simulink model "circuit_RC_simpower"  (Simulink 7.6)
settings: Solver=ode23t  StartTime=0.0  StopTime=0.04  RelTol=1e-3
InitFcn:
  | clc, close all
StopFcn:
  | close all
  | load tension_Vc.mat
  | plot(x(1,:),x(2,:), x(1,:),x(3,:),x(1,:),x(4,:))
  | axis([0 0.04 -60 120])
  | grid
  | title('Tension aux bornes de C, courant et créneau d''entrée')
  | xlabel('temps')
libraries: powerlib x9

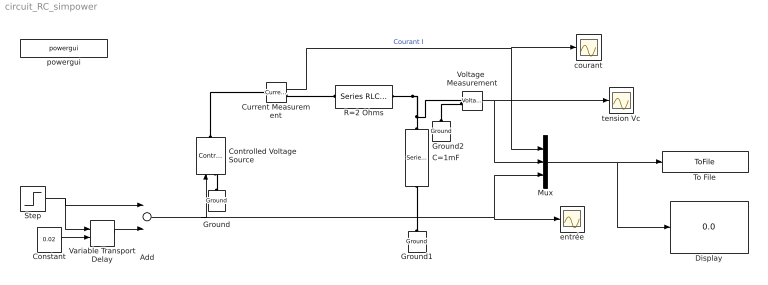
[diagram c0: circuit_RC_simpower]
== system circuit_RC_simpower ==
  Add : Sum  Inputs=+-
  C=1mF : powerlib/Elements/Series RLC Branch  DialogController=POWERSYS.PowerSysDialog  PhysicalDomain=powersysdomain  SubClassName=unknown  LeftPortType=p1  RightPortType=p1  LConnTagsString=__new0  RConnTagsString=__new0  BranchType=C  Resistance=2  Inductance=1e-3  SetiL0=off  InitialCurrent=0  Capacitance=1e-3  Setx0=off  InitialVoltage=0  Measurements=None
  Constant : Constant  Value=0.02
  Controlled Voltage Source : powerlib/Electrical Sources/Controlled Voltage Source  DialogController=POWERSYS.PowerSysDialog  SystemSampleTime=-1  Initialize=on  Source_Type=AC  Amplitude=0  Phase=0  Frequency=0  Measurements=None
  Current Measurement : powerlib/Measurements/Current Measurement  DialogController=POWERSYS.PowerSysDialog  SystemSampleTime=-1  PhasorSimulation=off  OutputType=Complex  PSBequivalent=0
  Display : Display
  Ground : powerlib/Elements/Ground  DialogController=POWERSYS.PowerSysDialog  PhysicalDomain=powersysdomain  SubClassName=unknown  LeftPortType=p1  RightPortType=p1  LConnTagsString=a
  Ground1 : powerlib/Elements/Ground  DialogController=POWERSYS.PowerSysDialog  PhysicalDomain=powersysdomain  SubClassName=unknown  LeftPortType=p1  RightPortType=p1  LConnTagsString=a
  Ground2 : powerlib/Elements/Ground  DialogController=POWERSYS.PowerSysDialog  PhysicalDomain=powersysdomain  SubClassName=unknown  LeftPortType=p1  RightPortType=p1  LConnTagsString=a
  Mux : Mux  Inputs=3
  R=2 Ohms : powerlib/Elements/Series RLC Branch  DialogController=POWERSYS.PowerSysDialog  PhysicalDomain=powersysdomain  SubClassName=unknown  LeftPortType=p1  RightPortType=p1  LConnTagsString=__new0  RConnTagsString=__new0  BranchType=R  Resistance=2  Inductance=1e-3  SetiL0=off  InitialCurrent=0  Capacitance=1e-6  Setx0=off  InitialVoltage=0  Measurements=None
  Step : Step  Time=0.005  After=100  SampleTime=0
  To File : ToFile  Filename=tension_Vc.mat  MatrixName=x
  Variable Transport Delay : VariableTransportDelay  VariableDelayType=Variable transport delay  MaximumDelay=10
  Voltage  Measurement : powerlib/Measurements/Voltage Measurement  DialogController=POWERSYS.PowerSysDialog  SystemSampleTime=-1  PhasorSimulation=off  OutputType=Complex  PSBequivalent=0
  courant : Scope
  entrée : Scope
  powergui : powerlib/powergui  Priority=1  SystemSampleTime=-1  SimulationMode=Continuous  SampleTime=50e-6  frequency=60  SPID=off  DisableSnubberDevices=off  DisableRonSwitches=off  DisableVfSwitches=off  SwTol=0  Interpol=off  frequencyindice=0  echomessages=off  HookPort=off  DisplayEquations=off  FunctionMessages=off  EnableUseOfTLC=off  x0status=blocks  RestoreLinks=warning  ResistiveCurrentMeasurement=off  Ylog=off  Xlog=on  ShowGrid=off  save=off  variable=ZData  ZoomFFT=off  StartTime=0.0  cycles=1  DisplayStyle=1  fundamental=60  FreqAxis=off  MaxFrequency=1000  frequencyindicesteady=1  display=off  methode=off
  tension Vc : Scope
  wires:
  Current Measurement/1 -> courant/1, Mux/1  "Courant I"
  Voltage  Measurement/1 -> tension Vc/1, Mux/2
  Mux/1 -> To File/1, Display/1
  Step/1 -> Add/1, Variable Transport Delay/1
  Variable Transport Delay/1 -> Add/2
  Add/1 -> Controlled Voltage Source/1, entrée/1, Mux/3
  Constant/1 -> Variable Transport Delay/2
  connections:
  Ground/LConn1 -- Controlled Voltage Source/LConn1
  Controlled Voltage Source/RConn1 -- Current Measurement/LConn1
  Current Measurement/RConn1 -- R=2 Ohms/LConn1
  Ground1/LConn1 -- C=1mF/RConn1
  Ground2/LConn1 -- Voltage  Measurement/LConn2
  C=1mF/LConn1 -- Voltage  Measurement/LConn1 -- R=2 Ohms/RConn1
